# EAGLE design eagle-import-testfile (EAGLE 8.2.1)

## Sheet 1 of 2: Sheet1
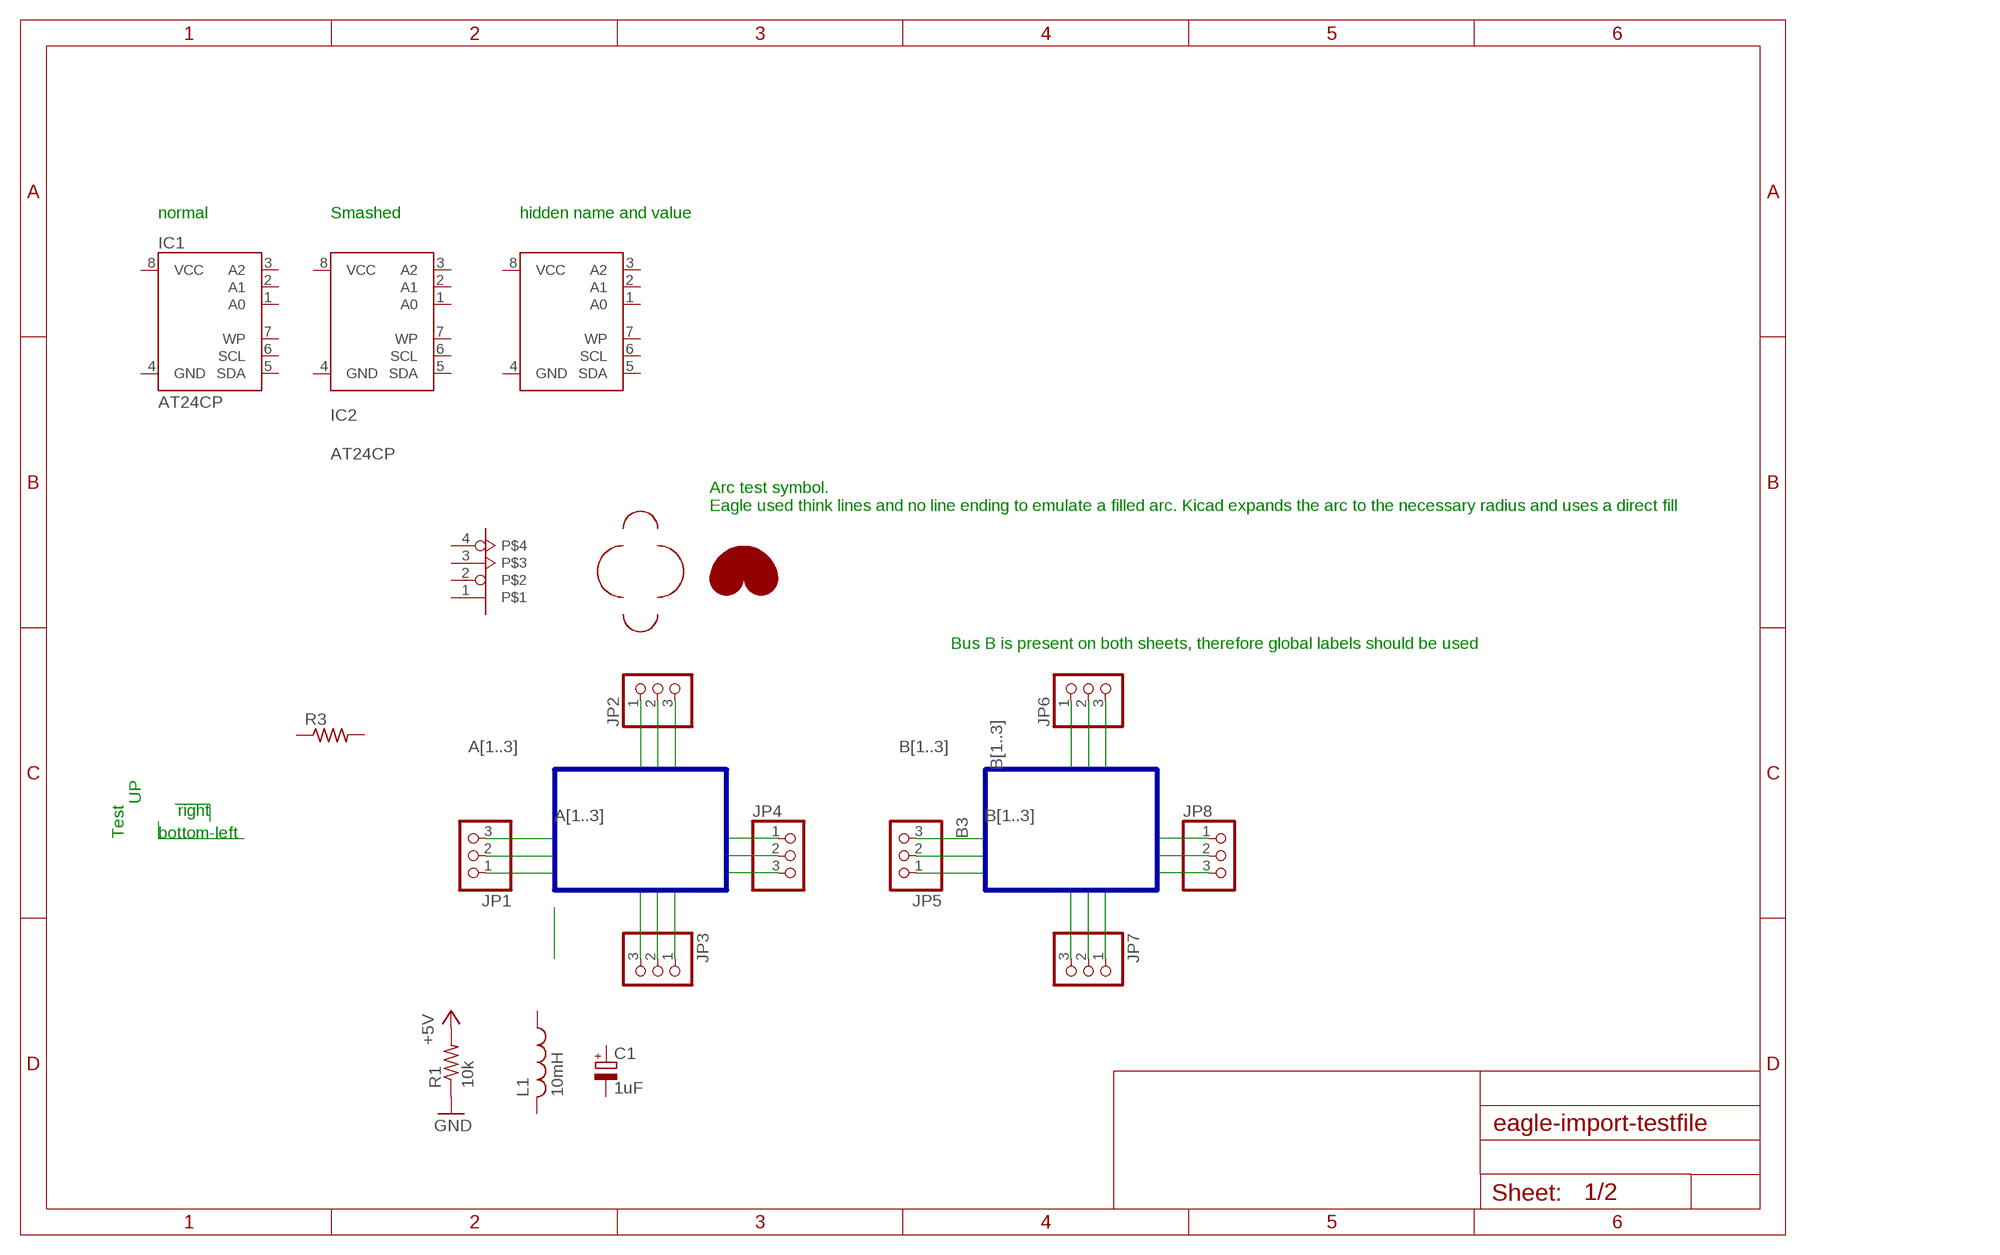
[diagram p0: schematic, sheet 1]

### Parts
C1  1uF  CPOL-EU085CS-1AR  [085CS_1AR]
IC1  AT24CP  [DIL08]
IC2  AT24CP  [DIL08]
IC3  AT24CP  [DIL08]
JP1  PINHD-1X3  [1X03]
JP2  PINHD-1X3  [1X03]
JP3  PINHD-1X3  [1X03]
JP4  PINHD-1X3  [1X03]
JP5  PINHD-1X3  [1X03]
JP6  PINHD-1X3  [1X03]
JP7  PINHD-1X3  [1X03]
JP8  PINHD-1X3  [1X03]
L1  10mH  L-USL2012C  [L2012C]
R1  10k  R-US_R0603  [R0603]
R3  R-US_0204/2V  [0204V]
U$2  PINSHAPETEST  [1X04]

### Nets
+5V: R1.2
A1: JP1.1 JP2.1 JP3.1 JP4.1
A2: JP1.2 JP2.2 JP3.2 JP4.2
A3: JP1.3 JP2.3 JP3.3 JP4.3
B1: JP5.1 JP6.1 JP7.3 JP8.1 ; also sheet 2
B2: JP5.2 JP6.2 JP7.2 JP8.2 ; also sheet 2
B3: JP5.3 JP6.3 JP7.1 JP8.3 ; also sheet 2
GND: R1.1
Unconnected: C1.+ C1.- IC1.1(A0) IC1.2(A1) IC1.3(A2) IC1.5(SDA) IC1.6(SCL) IC1.7(WP) IC2.1(A0) IC2.2(A1) IC2.3(A2) IC2.5(SDA) IC2.6(SCL) IC2.7(WP) IC3.1(A0) IC3.2(A1) IC3.3(A2) IC3.5(SDA) IC3.6(SCL) IC3.7(WP) L1.1 L1.2 R3.1 R3.2 U$2.1 U$2.2 U$2.3 U$2.4

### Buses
A[1..3]
B[1..3]

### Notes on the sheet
- normal | Smashed | hidden name and value
- Arc test symbol.
  Eagle used think lines and no line ending to emulate a filled arc. Kicad expands the arc to the necessary radius and uses a direct fill
- Bus B is present on both sheets, therefore global labels should be used
- UP | right
- Test | bottom-left

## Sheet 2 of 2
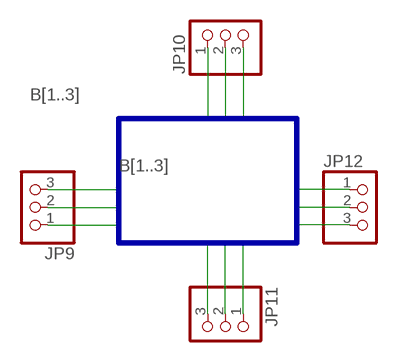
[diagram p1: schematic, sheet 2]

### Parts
JP9  PINHD-1X3  [1X03]
JP10  PINHD-1X3  [1X03]
JP11  PINHD-1X3  [1X03]
JP12  PINHD-1X3  [1X03]

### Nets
B1: JP9.1 JP10.1 JP11.3 JP12.1 ; also sheet 1
B2: JP9.2 JP10.2 JP11.2 JP12.2 ; also sheet 1
B3: JP9.3 JP10.3 JP11.1 JP12.3 ; also sheet 1

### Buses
B[1..3]

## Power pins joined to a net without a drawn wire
GND: IC1.4(GND) IC2.4(GND) IC3.4(GND)
VCC: IC1.8(VCC) IC2.8(VCC) IC3.8(VCC)

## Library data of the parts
C1 = rcl:CPOL-EU: POLARIZED CAPACITOR, European symbol
IC1-IC3 = atmel:AT24C*: 2-wire serial EEPROM; MPN: AT24C1024BW-SH-B; OC_FARNELL: 1362646; OC_NEWARK: 03P2044
JP1-JP12 = pinhead:PINHD-1X3: PIN HEADER
L1 = rcl:L-US: INDUCTOR, American symbol
R1 R3 = resistor:R-US_: RESISTOR, American symbol
U$2 = pinhead:PINSHAPETEST

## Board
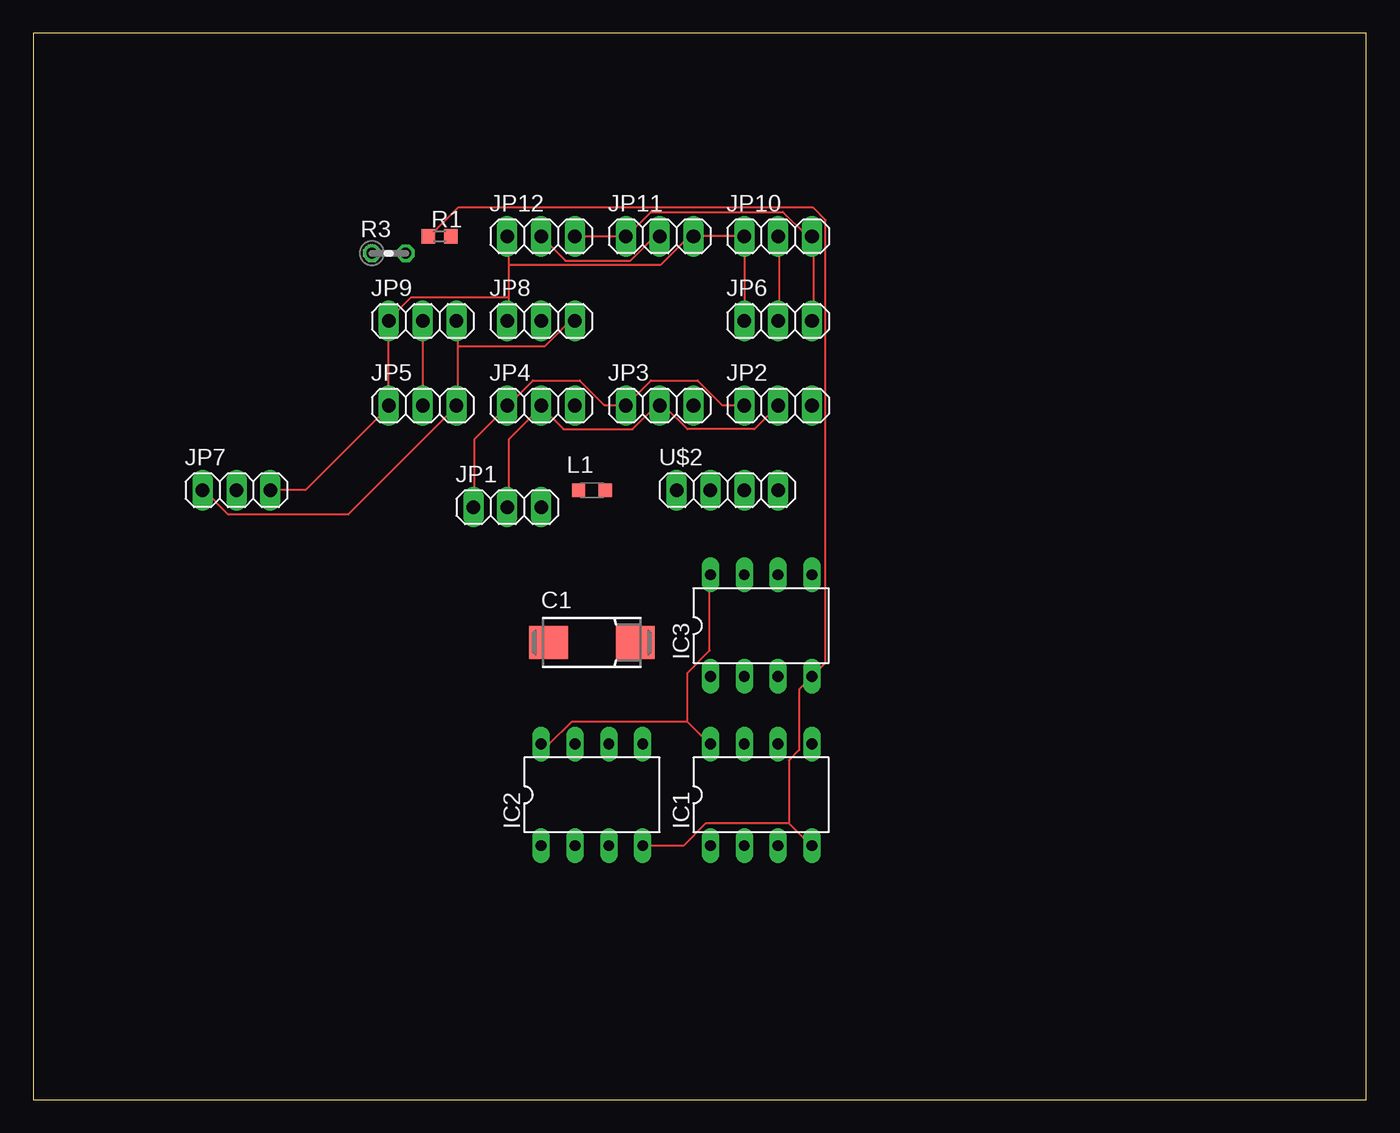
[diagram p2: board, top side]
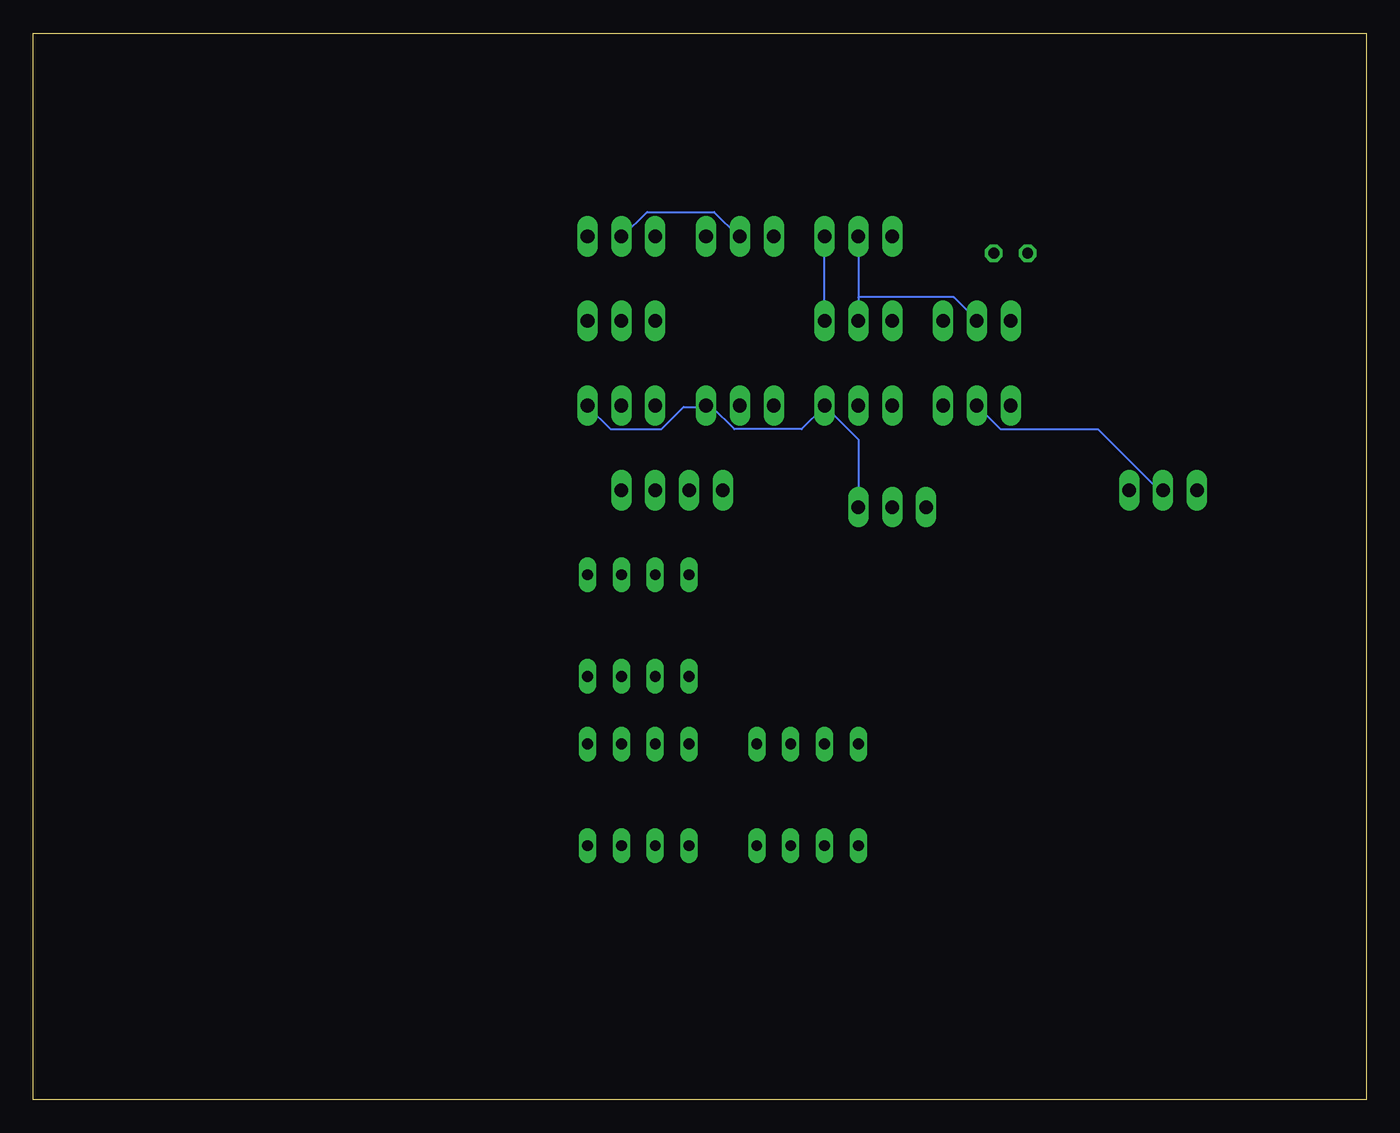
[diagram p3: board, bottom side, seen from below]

Size 100 x 80 mm. Coordinates in mm from the lower left corner, seen from the top.
Outline: 0,0 100,0 100,80 0,80 0,0
Copper layers (1*16): Top 0.035mm / dielectric 1.5mm / Bottom 0.035mm
Design rules "default": minimum track width 6mil, minimum drill 0.35mm, track to track 6mil, track to pad 6mil, pad to pad 6mil, via to via 6mil, smd to smd 6mil, copper to edge 40mil, drill to drill 6mil, minimum pad ring 10mil, minimum via ring 8mil, stop-mask expansion 4mil, vias tented up to drill 0mil, thermal gap 10mil

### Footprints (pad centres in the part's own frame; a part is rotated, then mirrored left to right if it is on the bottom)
085CS_1AR = smd 2.9 x 2.5: + 3.25,0; - -3.25,0
DIL08 = drill 0.813 long: 1 -3.81,-3.81; 2 -1.27,-3.81; 3 1.27,-3.81; 4 3.81,-3.81; 5 3.81,3.81; 6 1.27,3.81; 7 -1.27,3.81; 8 -3.81,3.81
1X03 = drill 1.016 long: 1 -2.54,0; 2 0,0; 3 2.54,0
L2012C = smd 1 x 1: 1 -1,0; 2 1,0
R0603 = smd 1 x 1.1: 1 -0.85,0; 2 0.85,0
0204V = drill 0.813 octagon: 1 -1.27,0; 2 1.27,0
1X04 = drill 1.016 long: 1 -3.81,0; 2 -1.27,0; 3 1.27,0; 4 3.81,0

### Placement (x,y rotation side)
C1  41.91,34.29 0 top
IC1  54.61,22.86 0 top
IC2  41.91,22.86 0 top
IC3  54.61,35.56 0 top
JP1  35.56,44.45 0 top
JP2  55.88,52.07 0 top
JP3  46.99,52.07 0 top
JP4  38.1,52.07 0 top
JP5  29.21,52.07 0 top
JP6  55.88,58.42 0 top
JP7  15.24,45.72 0 top
JP8  38.1,58.42 0 top
JP9  29.21,58.42 0 top
JP10  55.88,64.77 0 top
JP11  46.99,64.77 0 top
JP12  38.1,64.77 0 top
L1  41.91,45.72 0 top
R1  30.48,64.77 0 top
R3  26.67,63.5 0 top
U$2  52.07,45.72 0 top

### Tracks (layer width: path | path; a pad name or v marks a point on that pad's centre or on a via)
A1
  Top 0.152: JP1.1 33.07,44.5 33.07,49.53 35.51,51.97 JP4.1 35.66,52.12 37.49,53.95 41,53.95 42.82,52.12 44.35,52.12 JP3.1 46.33,53.95 49.84,53.95 51.66,52.12 53.34,52.12 JP2.1
A2
  Top 0.152: JP2.2 54.1,50.29 49.07,50.29 47.4,51.97 47.09,51.97 JP3.2 46.94,51.97 46.63,51.97 44.96,50.29 39.78,50.29 38.1,51.97 | 38.1,51.97 35.66,49.53 35.66,44.5 JP1.2 | 38.1,51.97 JP4.2
A3
  Bottom 0.152: 49.53,51.97 51.21,51.97 52.88,50.29 56.69,50.29 58.37,51.97 JP2.3 | JP1.3 38.1,49.53 JP4.3 40.69,51.97 42.37,50.29 47.4,50.29 49.07,51.97 49.53,51.97 | 49.53,51.97 JP3.3
B1
  Top 0.152: JP6.1 JP10.1 JP11.3 49.23,64.77 47.09,62.64 35.66,62.64 | 35.66,62.64 35.66,64.77 JP12.1 | 35.66,62.64 35.66,60.2 | 35.66,60.2 35.66,58.52 JP8.1 | JP7.3 20.42,45.72 26.67,51.97 JP5.1 JP9.1 26.67,58.52 28.35,60.2 35.66,60.2
B2
  Top 0.152: JP6.2 55.93,58.52 55.93,64.77 JP10.2 | JP9.2 29.26,58.37 29.26,52.12 JP5.2 | JP11.2 46.63,64.77 44.81,62.94 39.93,62.94 JP12.2
  Bottom 0.152: JP11.2 47.09,64.77 48.92,66.6 53.95,66.6 55.78,64.77 JP10.2 | JP12.2 38.1,60.2 | 38.1,60.2 JP8.2 | JP7.2 15.54,45.72 20.12,50.29 27.43,50.29 JP5.2 | 38.1,60.2 30.94,60.2 29.26,58.52 JP9.2
B3
  Top 0.152: JP6.3 58.52,58.52 58.52,64.77 JP10.3 58.06,64.77 56.24,66.6 46.33,66.6 44.5,64.77 JP11.1 JP12.3 | JP7.1 12.8,45.72 14.63,43.89 23.62,43.89 31.7,51.97 JP5.3 31.85,52.12 31.85,56.54 | 31.85,56.54 31.85,58.37 JP9.3 | 31.85,56.54 38.41,56.54 40.23,58.37 40.54,58.37 JP8.3
  Bottom 0.152: JP8.3 40.69,58.52 40.69,64.77 JP12.3
GND
  Top 0.152: IC2.4 48.77,19.05 50.44,20.73 56.69,20.73 | 56.69,20.73 58.37,19.05 IC1.4 | R1.1 29.72,64.77 31.85,66.9 58.52,66.9 59.44,65.99 59.44,32.77 IC3.4 57.45,30.79 57.45,26.21 56.69,25.45 56.69,20.73
VCC
  Top 0.152: IC2.8 38.71,26.67 40.39,28.35 49.07,28.35 | 49.07,28.35 50.75,26.67 IC1.8 | 49.07,28.35 49.07,32 50.75,33.68 50.75,39.32 IC3.8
